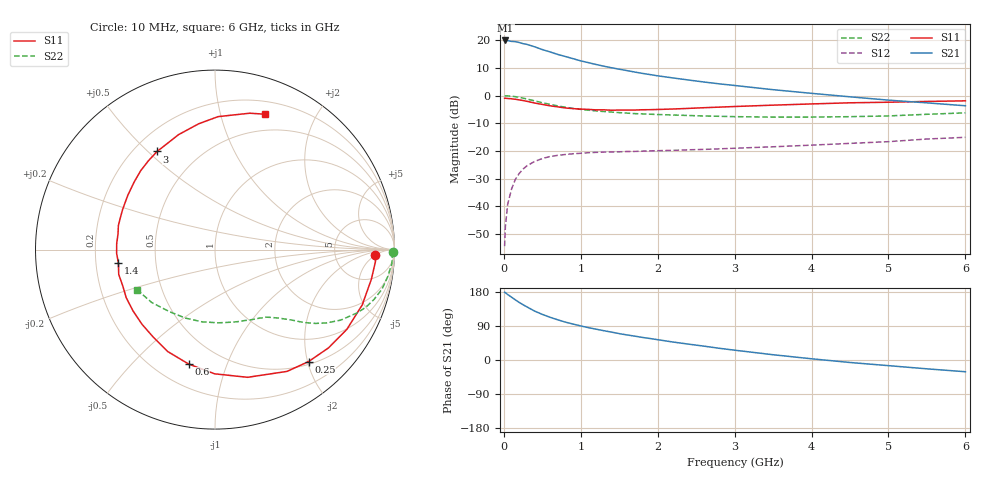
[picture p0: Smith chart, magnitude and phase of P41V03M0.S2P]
! SIEMENS Small Signal Semiconductors
! BFP182
! Si NPN RF Bipolar Junction Transistor in SOT143
! VCE = 1 V  IC = 3 mA
! Common Emitter S-Parameters:  March  1996
# GHz  S  MA  R  50
!  f  S11  S21  S12  S22
! GHz  MAG  ANG  MAG  ANG  MAG  ANG  MAG  ANG
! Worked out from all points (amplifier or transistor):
!   36 points, 10 MHz to 6 GHz, reference 50 ohm
!   highest |S21| = 19.9 dB at 20 MHz (marker M1)
!   |S21| within 3 dB of that: start of sweep to 470.4 MHz
!   unconditionally stable (mu >= 1): 1.827 GHz to end of sweep
!   at 250 MHz: K = 0.16, MSG = 22.7 dB, |S12| = -26.6 dB
!   at 1.4 GHz: K = 0.81, MSG = 15.2 dB, |S12| = -20.3 dB
!   at 6 GHz: K = 1.04, MAG = 4.5 dB, |S12| = -15.1 dB
!   S11 on the Smith chart (normalised r, x): 10 MHz: 16, -5; 250 MHz: 0.55, -2.02; 600 MHz: 0.33, -0.74; 1.4 GHz: 0.30, -0.06; 3 GHz: 0.29, +0.53; 6 GHz: 0.32, +1.38
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0.01  0.8927 -2.1  9.708 178.9  0.0019 89.8  0.9925 -0.9
0.02  0.8964 -4.3  9.918 177.7  0.0043 91.9  0.9885 -1.8
0.05  0.8868 -10.7  9.845 172.7  0.0109 86.3  0.9887 -4.5
0.15  0.8585 -31.2  9.434 158.7  0.0306 71.7  0.9562 -13.3
0.2  0.8365 -40.9  9.111 151.9  0.0392 67.7  0.9292 -17.3
0.25  0.813 -50.1  8.687 145.8  0.0469 62.9  0.9007 -20.8
0.3  0.7884 -59.4  8.424 140.2  0.0539 58.1  0.8679 -23.9
0.4  0.7343 -75.7  7.621 129.1  0.0645 50.5  0.803 -29.3
0.5  0.692 -90.2  6.784 120.4  0.0729 44.0  0.7439 -33.3
0.6  0.6542 -103.0  6.163 112.8  0.0792 39.3  0.6948 -36.3
0.7  0.626 -114.9  5.548 106.1  0.0832 35.5  0.6518 -38.7
0.8  0.597 -125.1  5.084 100.0  0.0862 32.3  0.6163 -40.6
0.9  0.5818 -134.4  4.646 94.8  0.0889 29.8  0.5862 -42.2
1.1  0.5625 -151.6  3.938 85.3  0.0929 26.0  0.5449 -45.1
1.4  0.5434 -172.0  3.184 73.6  0.0961 21.8  0.5038 -48.9
1.8  0.5547 166.0  2.523 59.6  0.099 20.2  0.4669 -54.0
2.2  0.5722 148.1  2.084 47.4  0.1024 19.0  0.4455 -60.4
3  0.6348 120.5  1.523 25.9  0.1117 18.3  0.4164 -75.9
3.5  0.6719 107.6  1.279 13.9  0.1188 17.8  0.4084 -87.4
4.5  0.7409 88.7  0.95 -6.6  0.1369 16.0  0.4159 -113.5
5.5  0.7841 75.7  0.739 -23.3  0.1641 13.1  0.4593 -140.0
6  0.804 69.8  0.655 -31.0  0.1762 9.5  0.4878 -152.5
